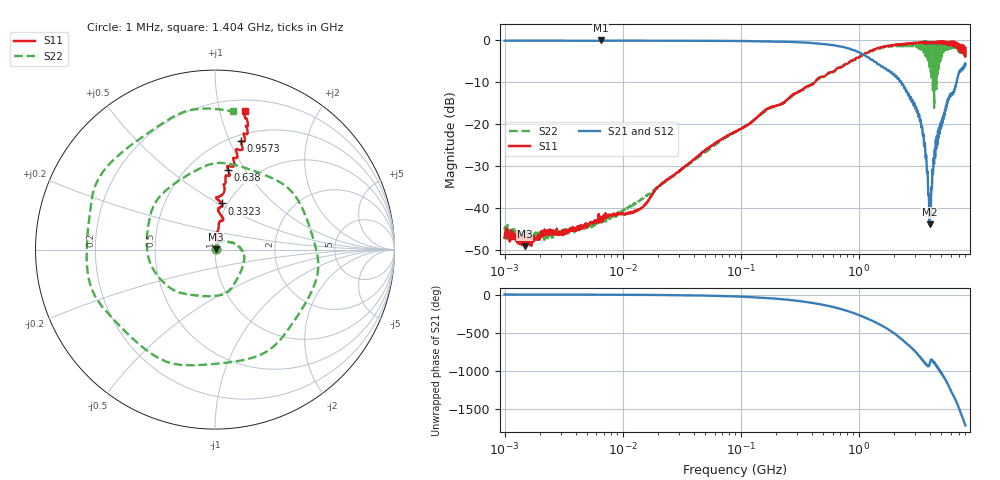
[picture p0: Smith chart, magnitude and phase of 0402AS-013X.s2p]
!s-Parameter Generated by FASTRON Sdn. Bhd.
!FASTRON P/N : 0402AS-013X
!Keysight Technologies: E5071C_MY46733604_B.14.02
!Date: Mon Dec 01 10:31:00 2025
!Version  :Rev00  Mon Dec 01 10:31:00 2025
!Data & Calibration Information:
!Freq  S11:SOLT2(ON)  S21:SOLT2(ON)  S12:SOLT2(ON)  S22:SOLT2(ON)
!PortZ  Port1:50+j0  Port2:50+j0
!When reading reference impedance value at option line is always used.
! Remarks : This data is being provided solely for informational purposes.
# Hz S dB R 50
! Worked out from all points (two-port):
!   1601 points, 1 MHz to 8 GHz, reference 50 ohm
!   highest |S21| = 0.01 dB at 6.532 MHz (marker M1); lowest = -43.9 dB at 3.974 GHz (marker M2)
!   |S21| within 3 dB of the highest: start of sweep to 1.036 GHz
!   lowest |S11| = -49.1 dB at 1.477 MHz (marker M3), VSWR 1.01, Z = 50.3 + j0.17 ohm
!   |S11| at or under -10 dB: start of sweep to 422 MHz
!   |S22| runs from -48.1 to -0.2 dB; largest |S21 - S12| = 0.016
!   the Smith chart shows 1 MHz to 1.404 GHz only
!   S11 on the Smith chart (normalised r, x): 1 MHz: 1.01, +0.00; 332.3 MHz: 0.94, +0.52; 638 MHz: 0.76, +0.84; 957.3 MHz: 0.56, +1.10; 1.404 GHz: 0.29, +1.20
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1000000  -47.10 16.7  -0.06 -0.3  -0.04 -0.3  -45.20 18.7
1477369  -49.10 28.8  -0.05 -0.4  -0.05 -0.4  -46.80 1.6
4479405  -44.20 41.1  -0.05 -1.2  -0.04 -1.3  -44.90 44.5
6531720  -43.30 43.6  0.01 -1.9  -0.02 -2.0  -43.20 52.9
2.00676e7  -34.90 63.4  -0.06 -5.6  -0.06 -5.5  -34.90 68.6
8.994653e7  -21.80 85.8  -0.12 -24.8  -0.12 -24.8  -21.90 32.7
3.322712e8  -11.70 81.4  -0.46 -90.2  -0.45 -90.2  -11.80 -86.5
4.006501e8  -10.60 85.6  -0.59 -109.0  -0.58 -109.0  -10.40 -126.0
6.379863e8  -6.96 80.5  -1.21 -172.0  -1.20 -172.0  -7.18 114.0
9.573479e8  -4.12 76.8  -2.60 103.0  -2.59 103.0  -4.23 -51.9
1.202604e9  -2.87 75.2  -3.98 40.7  -3.98 40.6  -2.89 -176.0
1.403687e9  -2.03 77.8  -5.20 -8.3  -5.19 -8.4  -2.20 82.4
1.581568e9  -1.67 80.8  -6.23 -49.5  -6.24 -49.7  -1.59 -2.7
1.7949e9  -1.31 85.2  -7.08 -101.0  -7.09 -101.0  -1.50 -109.0
2.103821e9  -0.97 90.9  -8.70 -177.0  -8.70 -177.0  -1.38 92.1
2.457552e9  -0.95 94.3  -11.30 99.9  -11.20 99.8  -0.90 -76.1
2.648292e9  -0.88 98.7  -12.90 57.0  -12.90 56.8  -0.72 -168.0
2.839031e9  -0.77 103.0  -14.50 14.4  -14.50 14.2  -0.57 102.0
3.183204e9  -0.49 111.0  -17.60 -71.4  -17.60 -71.8  -1.37 -85.3
3.568312e9  -0.32 122.0  -24.60 -166.0  -24.60 -166.0  -2.36 63.8
3.973689e9  -0.48 126.0  -43.90 164.0  -43.80 164.0  -3.18 -130.0
8e9  -1.83 -111.0  -5.77 85.5  -5.80 85.1  -3.60 119.0
